(* Logix 5000 AddOnInstructionDefinition export Banner_K50Audible_Param_v4; software revision 32.00 *)

TYPE Banner_IOL_Port_v4 :   // UDT that has all of the data items necessary to communicate with a specific Port on a IO-Link Master
STRUCT
   Port_Controlled : INT;   // Each bit represents a port on an IO-Link Master. Set to 1 to tell AOI to control that port.
   Port_Activate : INT;   // Each bit represents a port on an IO-Link Master. When ON that port will process any commands in queue.
   Port_Read : INT;   // Each bit represents a port on an IO-Link Master. Used to determine when device AOI has requested a Read command.
   Port_Write : INT;   // Each bit represents a port on an IO-Link Master. Used to determine when device AOI has requested a Write command.
   Port_RW_Complete : INT;   // Each bit represents a port on an IO-Link Master. Tells device AOI that Read or Write request has been completed.
   Port_Device_Read : INT;
   Data_Transfer : SINT[190];   // Array to transfer data from IO-Master to device AOIs.
END_STRUCT
END_TYPE

TYPE Banner_K50Audible_RD_v2 :   // UDT with all of the Read only parameters for K50 Pro Audible.
STRUCT
   Master_Cycle_Time : INT;
   Min_Cycle_Time : INT;
   M_Sequence_Capability : INT;
   IO_Link_Version_ID : INT;
   Process_Data_Input_Length : INT;
   Process_Data_Output_Length : INT;
   Combined_Vendor_ID : DINT;   // IO-Link Vendor ID
   Vendor_ID1 : INT;
   Vendor_ID2 : INT;
   Combined_Device_ID : DINT;   // IO-Link Device ID
   Device_ID1 : INT;
   Device_ID2 : INT;
   Device_ID3 : INT;
   Serial_Number : STRING;
END_STRUCT
END_TYPE

TYPE Banner_K50Audible_SP_v2 :   // UDT for K50 Pro Audible Touch with the State Parameters structure.
STRUCT
   Type : SINT;   // 0 = Off, 1 = Steady, 2 = Flash, 3 = Two Color Flash, 4 = 50/50, 5 = 50/50 Rotate, 6 = Chase, 7 = Intensity Sweep, 8 = Sequence.
   Direction : SINT;   // 0 = CCW, 1 = CW.
   Pattern : SINT;   // 0 = Flash, 1 = Strobe, 2 = Three Pulse, 3 = SOS, 4 = Random.
   Speed : SINT;   // 0 = Slow, 1 = Medium, 2 = Fast, 3 = Custom.
   Audio_Feedback : SINT;   // 0 = Off, 1 = On, 2 = Animation Pattern, 3 = Advanced Audible
   Off_Delay_Type : SINT;   // 0 =Leading Edge, 1 = Trailing Edge.
   Off_Delay : DINT;   // 0 to 65535 in ms. Length of time before the device returns to 'touch inactive' state after button is released.
   Static_Sequence : INT;   // 0 to 255. Value describing the LED position of the device.
   Sequence_Start_Location : SINT;   // 0 = LED1, 1 = LED2, 2 = LED3, 3 = LED4, 4 = LED5, 5 = LED6, 6 = LED7, 7 = LED8.
   Color_1 : SINT;   // 0 = Green, 1 = Red, 2 = Orange, 3 = Amber, 4 = Yellow, 5 = Lime Green, 6 = Spring Green, 7 = Cyan, 8 = SKy Blue, 9 = Blue, 10 = Violet, 11 = Magenta, 12 = Rose, 13 = White, 14 Custom 1, 15 = Custom 2.
   Color_1_Intensity : SINT;   // 0 = High, 1 = Medium, 2 = Low, 3 = Off, 4 = Custom.
   Color_2 : SINT;   // 0 = Green, 1 = Red, 2 = Orange, 3 = Amber, 4 = Yellow, 5 = Lime Green, 6 = Spring Green, 7 = Cyan, 8 = SKy Blue, 9 = Blue, 10 = Violet, 11 = Magenta, 12 = Rose, 13 = White, 14 Custom 1, 15 = Custom 2.
   Color_2_Intensity : SINT;   // 0 = High, 1 = Medium, 2 = Low, 3 = Off, 4 = Custom.
   Audio_Volume : SINT;   // 1 = Low, 3 = High
   Audio_Type : SINT;   // 0 = Pulse, 1 = Wobble, 2 = Strobe, 3 = Whoop, 4 = Stacatto, 5 = Siren, 6 = Continuous 1, 7 = Continuous 2, 9 = Jingle, 10 = Melody 1, 11 = Melody 2, 12 = Melody 3, 13 = Custom
END_STRUCT
END_TYPE

TYPE Banner_K50Audible_v2 :   // UDT with all of the parameters for K50 Pro Audible.
STRUCT
   Initial_Global_Read : BOOL;   // Determines if all of the IO-Link data has been read into the PLC yet
   Command : INT;   // Value placed in here will activate a read or write to a specifc IO-Link Index
   Read_Data : Banner_K50Audible_RD_v2;   // All read data
   Write_Data : Banner_K50Audible_WD_v2;   // All data that can be written to.
   Archive : Banner_K50Audible_WD_v2;   // Archive of the write data.
   Reset : BOOL;
END_STRUCT
END_TYPE

TYPE Banner_K50Audible_WD_v2 :   // UDT that stores the Write Data for a K50 Pro Audible.
STRUCT
   System_Command : INT;   // See IODD file for list of commands that can be activated via the System Command interface
   Parameter_Access_Lock : SINT;   // Write access to all read/write parameters is block when this bit is ON.
   Data_Storage_Lock : SINT;   // Data storage mechanism is inhibited when bit is ON.
   Local_Parameterization_Lock : SINT;   // Parameteriation via local control elementes is inhibited.
   Local_User_Interface_Lock : SINT;   // Operation of the hmi on the device is disabled.
   Operation_Mode : SINT;   // 0 = Multicolor, 1 = Four State Full Logic, 2 = Advanced, 3 = LED Control, 4 = Demo.
   Custom_Intensity : SINT;   // 0 to 100 %
   Custom_Flash_Rate : INT;   // Range 5 to 200 (.5 to 20 converted rate).
   Restrict_to_Gamut : SINT;   // 0 = Off, 1 = On.
   Touch_Sensitivity : SINT;   // 0 = Low, 1 = High.
   Function : SINT;   // 0 = Momentary, 1 = Latched.
   Mute_Enable : SINT;   // 0 = Off, 1 = On.
   On_Delay : DINT;   // 0 to 65535 in ms. Length of time the touch button needs to be pressed to trigger touch active state.
   Output_State : SINT;   // 0 = NO, 1 = NC.
   Off_Delay_Type : SINT;   // 0 = Leading Edge, 1 = Trailing Edge.
   Off_Delay : DINT;   // 0 to 65535 in ms. Length of time before the device returns to the 'touch inactive' state after button is released.
   State_Parameters : Banner_K50Audible_SP_v2[5];   // State Parameters. 1 through 4 will have values.
   CC1_Red : INT;   // 0-255. Custom 1 Red.
   CC1_Green : INT;   // 0-255. Custom 1 Green.
   CC1_Blue : INT;   // 0-255. Custom 1 Blue.
   CC2_Red : INT;   // 0-255. Custom 2 Red.
   CC2_Green : INT;   // 0-255. Custom 2 Green.
   CC2_Blue : INT;   // 0-255. Custom 2 Blue.
   Audio_Type : SINT;   // 0 = Beep, 1 = Sweep, 2 = Tone
   Sweep_Type : SINT;   // 0 = Up, 1 = Down, 2 = Up Down, 3 = Down Up
   Freq_1 : SINT;   // 0 = Off, 1 = Low, 2 = Standard, 3 = High
   Freq_2 : SINT;   // 0 = Off, 1 = Low, 2 = Standard, 3 = High
END_STRUCT
END_TYPE

ADD_ON_INSTRUCTION Banner_K50Audible_Param_v4   (* revision 4.0, vendor Banner Engineering *)
// AOI to read and write parameter data to an IO-Link K50 Pro Audible.
VAR_IN_OUT
   K50 : Banner_K50Audible_v2; {required}
   Port_Data : Banner_IOL_Port_v4; {required}
END_VAR
VAR_INPUT
   Port : DINT; {required}
END_VAR
VAR
   Local_Control : DINT; {access None}
   Global_Read_Command_Value : INT; {access None}
   Global_Write_Command_Value : INT; {access None}
   Command_Being_Processed : BOOL; {access None}
   Update_Archive : BOOL; {access None}
   Index_Write_Control : DINT; {access None}
   Index_Write_Inprocess : INT; {access None}
   Temp_Excess_Gain : DINT[2]; {access None}
   Inprocess_Index : DINT; {access None}
   SP_Index : DINT; {access None}   // State Parameters Index
   SP_Write_Index : DINT; {access None}
   SP_R_Index : DINT; {access None}
   SP_W_Index : DINT; {access None}
END_VAR

ROUTINE Logic   (* ladder *)
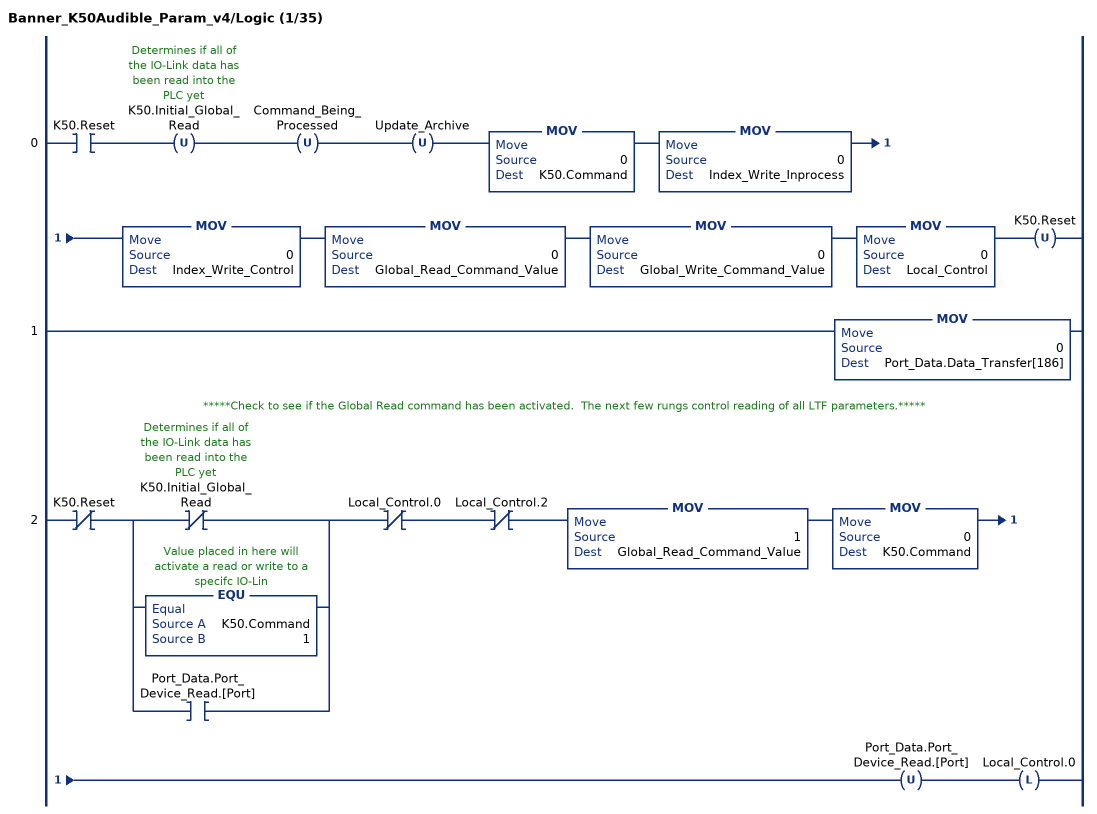
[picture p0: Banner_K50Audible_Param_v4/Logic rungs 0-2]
   0: XIC(K50.Reset)OTU(K50.Initial_Global_Read)OTU(Command_Being_Processed)OTU(Update_Archive)MOV(0,K50.Command)MOV(0,Index_Write_Inprocess)MOV(0,Index_Write_Control)MOV(0,Global_Read_Command_Value)MOV(0,Global_Write_Command_Value)MOV(0,Local_Control)OTU(K50.Reset);
   1: MOV(0,Port_Data.Data_Transfer[186]);
   // *****Check to see if the Global Read command has been activated.  The next few rungs control reading of all LTF parameters.*****
   2: XIO(K50.Reset)[XIO(K50.Initial_Global_Read) ,EQU(K50.Command,1) ,XIC(Port_Data.Port_Device_Read.[Port]) ]XIO(Local_Control.0)XIO(Local_Control.2)MOV(1,Global_Read_Command_Value)MOV(0,K50.Command)OTU(Port_Data.Port_Device_Read.[Port])OTL(Local_Control.0);
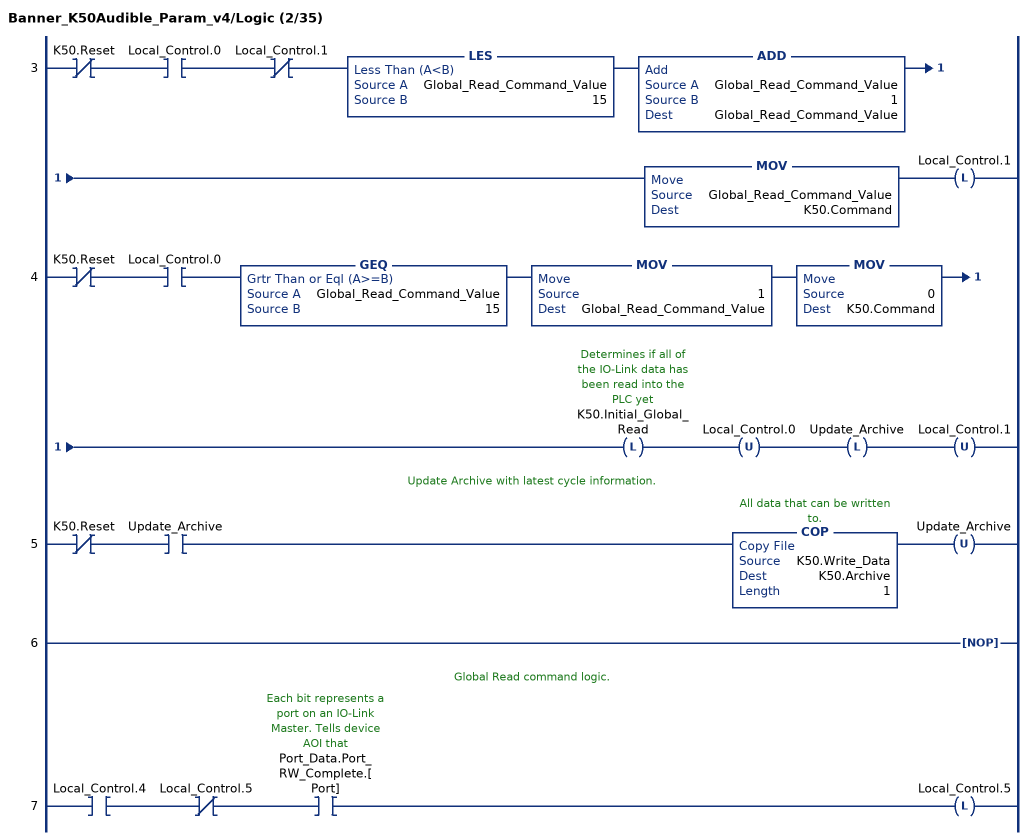
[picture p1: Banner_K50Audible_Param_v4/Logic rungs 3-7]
   3: XIO(K50.Reset)XIC(Local_Control.0)XIO(Local_Control.1)LES(Global_Read_Command_Value,15)ADD(Global_Read_Command_Value,1,Global_Read_Command_Value)MOV(Global_Read_Command_Value,K50.Command)OTL(Local_Control.1);
   4: XIO(K50.Reset)XIC(Local_Control.0)GEQ(Global_Read_Command_Value,15)MOV(1,Global_Read_Command_Value)MOV(0,K50.Command)OTL(K50.Initial_Global_Read)OTU(Local_Control.0)OTL(Update_Archive)OTU(Local_Control.1);
   // Update Archive with latest cycle information.
   5: XIO(K50.Reset)XIC(Update_Archive)COP(K50.Write_Data,K50.Archive,1)OTU(Update_Archive);
   6: NOP();
   // Global Read command logic.
   7: XIC(Local_Control.4)XIO(Local_Control.5)XIC(Port_Data.Port_RW_Complete.[Port])OTL(Local_Control.5);
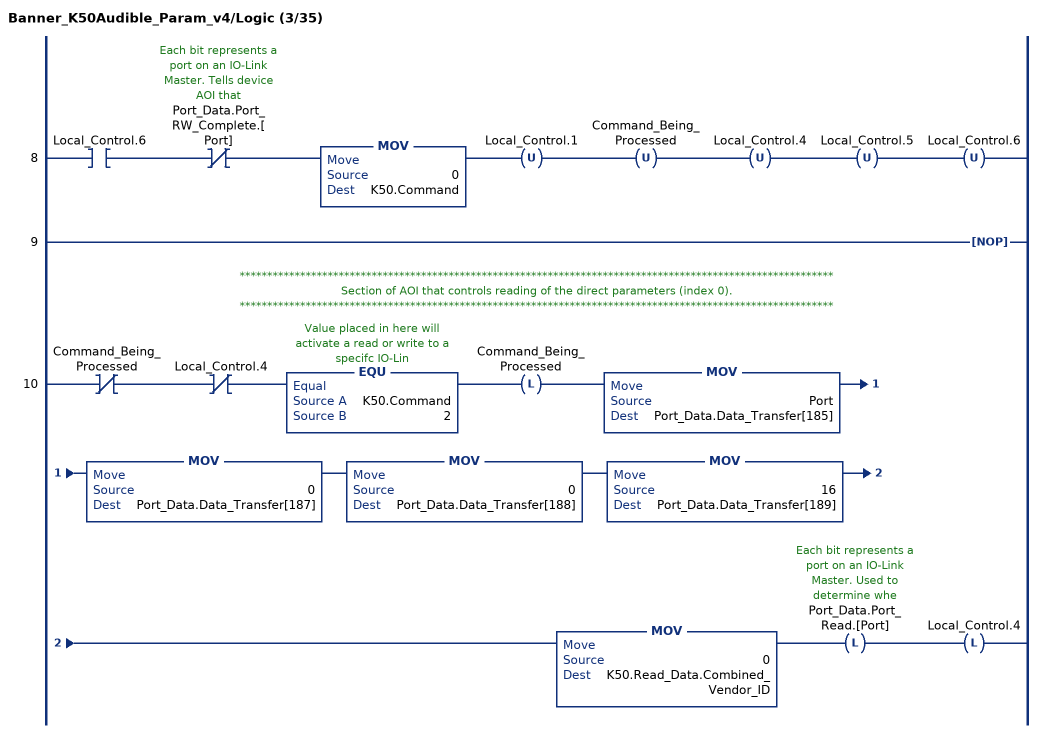
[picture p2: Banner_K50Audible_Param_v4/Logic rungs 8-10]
   8: XIC(Local_Control.6)XIO(Port_Data.Port_RW_Complete.[Port])MOV(0,K50.Command)OTU(Local_Control.1)OTU(Command_Being_Processed)OTU(Local_Control.4)OTU(Local_Control.5)OTU(Local_Control.6);
   9: NOP();
   // ************************************************************************************************************
   // Section of AOI that controls reading of the direct parameters (index 0).
   // ************************************************************************************************************
   10: XIO(Command_Being_Processed)XIO(Local_Control.4)EQU(K50.Command,2)OTL(Command_Being_Processed)MOV(Port,Port_Data.Data_Transfer[185])MOV(0,Port_Data.Data_Transfer[187])MOV(0,Port_Data.Data_Transfer[188])MOV(16,Port_Data.Data_Transfer[189])MOV(0,K50.Read_Data.Combined_Vendor_ID)OTL(Port_Data.Port_Read.[Port])OTL(Local_Control.4);
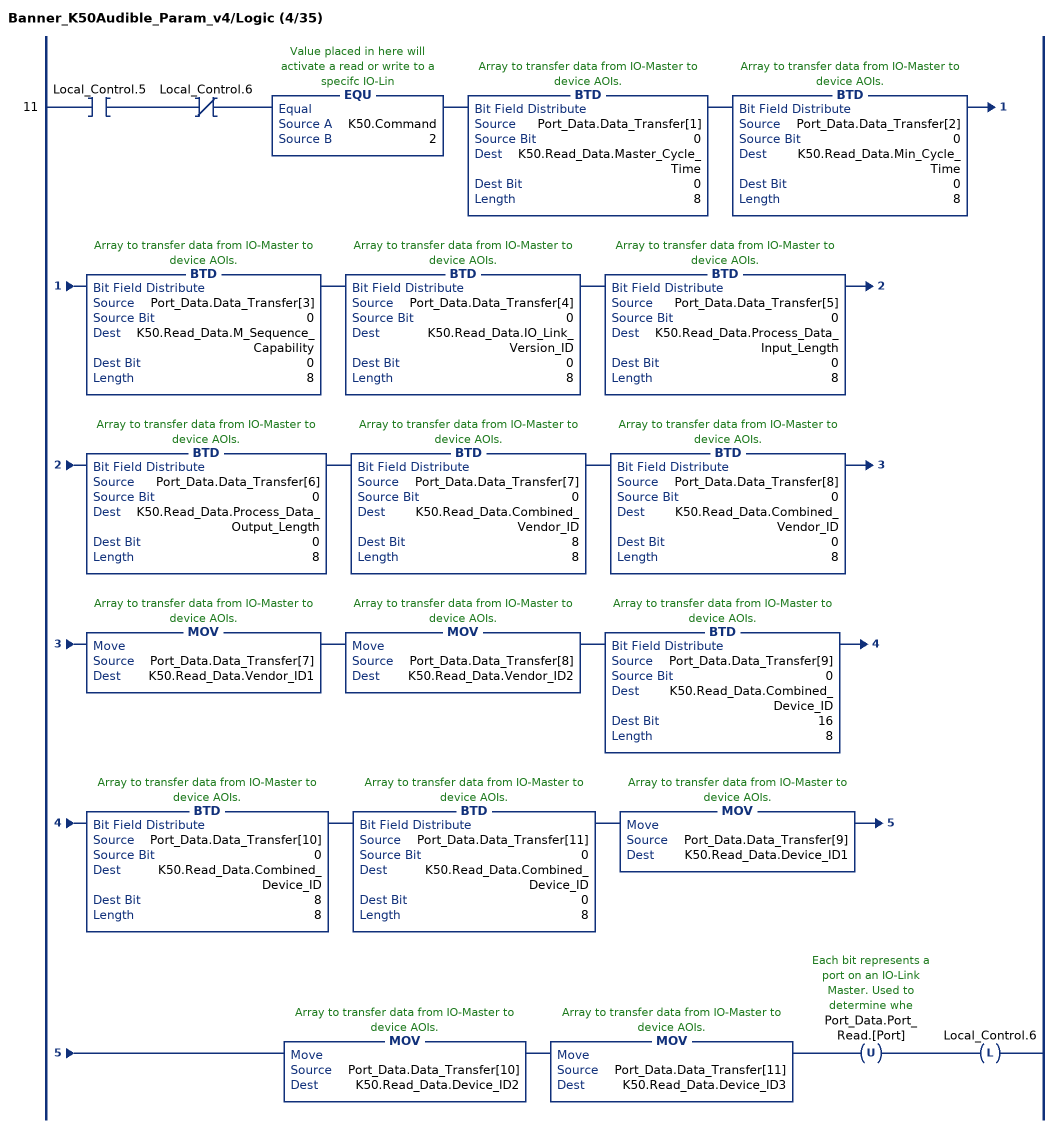
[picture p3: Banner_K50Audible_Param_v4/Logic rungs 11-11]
   11: XIC(Local_Control.5)XIO(Local_Control.6)EQU(K50.Command,2)BTD(Port_Data.Data_Transfer[1],0,K50.Read_Data.Master_Cycle_Time,0,8)BTD(Port_Data.Data_Transfer[2],0,K50.Read_Data.Min_Cycle_Time,0,8)BTD(Port_Data.Data_Transfer[3],0,K50.Read_Data.M_Sequence_Capability,0,8)BTD(Port_Data.Data_Transfer[4],0,K50.Read_Data.IO_Link_Version_ID,0,8)BTD(Port_Data.Data_Transfer[5],0,K50.Read_Data.Process_Data_Input_Length,0,8)BTD(Port_Data.Data_Transfer[6],0,K50.Read_Data.Process_Data_Output_Length,0,8)BTD(Port_Data.Data_Transfer[7],0,K50.Read_Data.Combined_Vendor_ID,8,8)BTD(Port_Data.Data_Transfer[8],0,K50.Read_Data.Combined_Vendor_ID,0,8)MOV(Port_Data.Data_Transfer[7],K50.Read_Data.Vendor_ID1)MOV(Port_Data.Data_Transfer[8],K50.Read_Data.Vendor_ID2)BTD(Port_Data.Data_Transfer[9],0,K50.Read_Data.Combined_Device_ID,16,8)BTD(Port_Data.Data_Transfer[10],0,K50.Read_Data.Combined_Device_ID,8,8)BTD(Port_Data.Data_Transfer[11],0,K50.Read_Data.Combined_Device_ID,0,8)MOV(Port_Data.Data_Transfer[9],K50.Read_Data.Device_ID1)MOV(Port_Data.Data_Transfer[10],K50.Read_Data.Device_ID2)MOV(Port_Data.Data_Transfer[11],K50.Read_Data.Device_ID3)OTU(Port_Data.Port_Read.[Port])OTL(Local_Control.6);
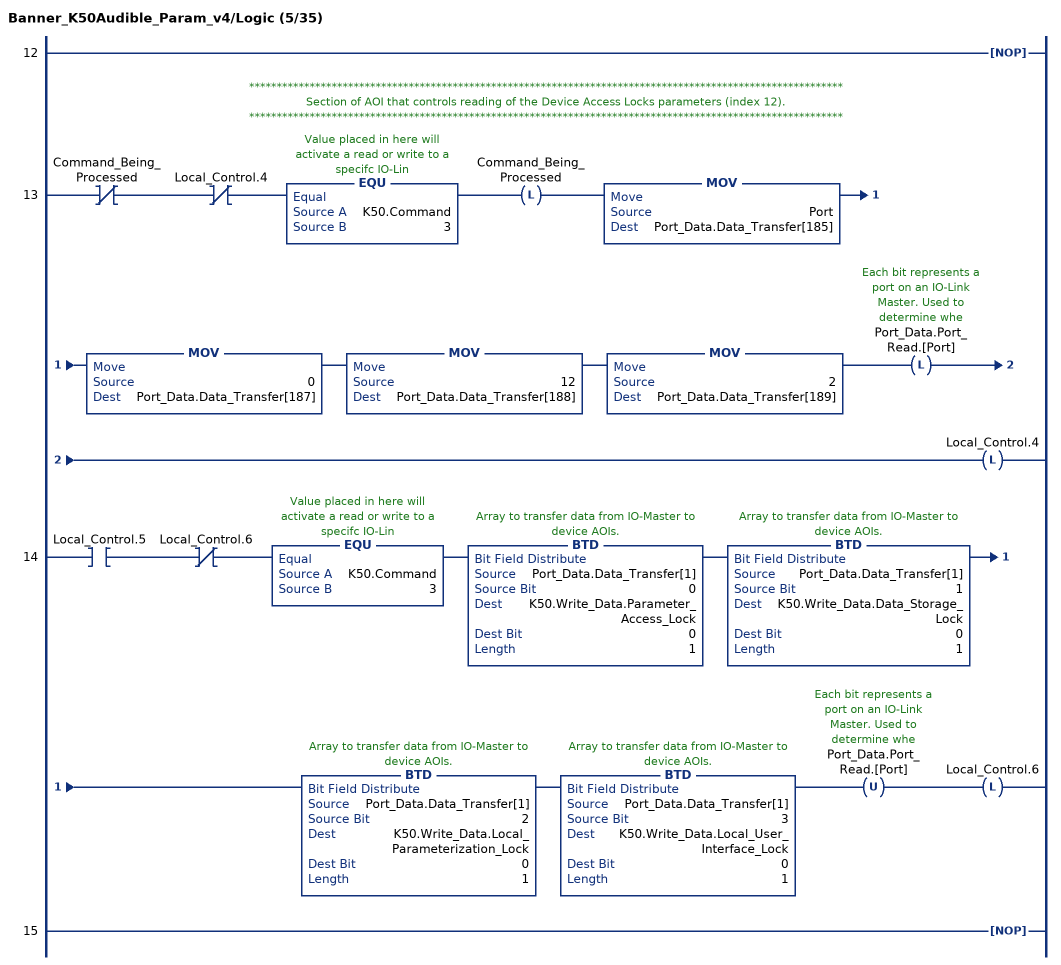
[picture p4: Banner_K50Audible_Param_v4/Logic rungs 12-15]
   12: NOP();
   // ************************************************************************************************************
   // Section of AOI that controls reading of the Device Access Locks parameters (index 12).
   // ************************************************************************************************************
   13: XIO(Command_Being_Processed)XIO(Local_Control.4)EQU(K50.Command,3)OTL(Command_Being_Processed)MOV(Port,Port_Data.Data_Transfer[185])MOV(0,Port_Data.Data_Transfer[187])MOV(12,Port_Data.Data_Transfer[188])MOV(2,Port_Data.Data_Transfer[189])OTL(Port_Data.Port_Read.[Port])OTL(Local_Control.4);
   14: XIC(Local_Control.5)XIO(Local_Control.6)EQU(K50.Command,3)BTD(Port_Data.Data_Transfer[1],0,K50.Write_Data.Parameter_Access_Lock,0,1)BTD(Port_Data.Data_Transfer[1],1,K50.Write_Data.Data_Storage_Lock,0,1)BTD(Port_Data.Data_Transfer[1],2,K50.Write_Data.Local_Parameterization_Lock,0,1)BTD(Port_Data.Data_Transfer[1],3,K50.Write_Data.Local_User_Interface_Lock,0,1)OTU(Port_Data.Port_Read.[Port])OTL(Local_Control.6);
   15: NOP();
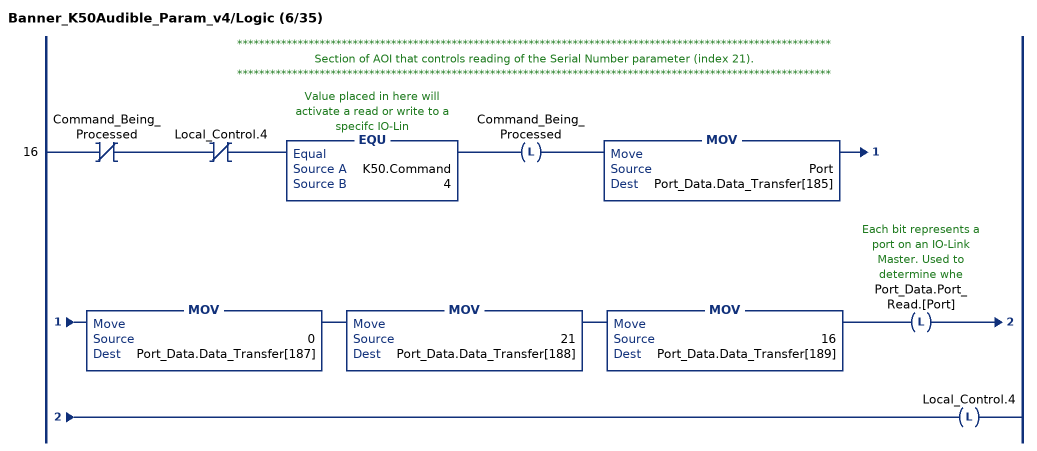
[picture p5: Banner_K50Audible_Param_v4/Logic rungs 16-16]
   // ************************************************************************************************************
   // Section of AOI that controls reading of the Serial Number parameter (index 21).
   // ************************************************************************************************************
   16: XIO(Command_Being_Processed)XIO(Local_Control.4)EQU(K50.Command,4)OTL(Command_Being_Processed)MOV(Port,Port_Data.Data_Transfer[185])MOV(0,Port_Data.Data_Transfer[187])MOV(21,Port_Data.Data_Transfer[188])MOV(16,Port_Data.Data_Transfer[189])OTL(Port_Data.Port_Read.[Port])OTL(Local_Control.4);
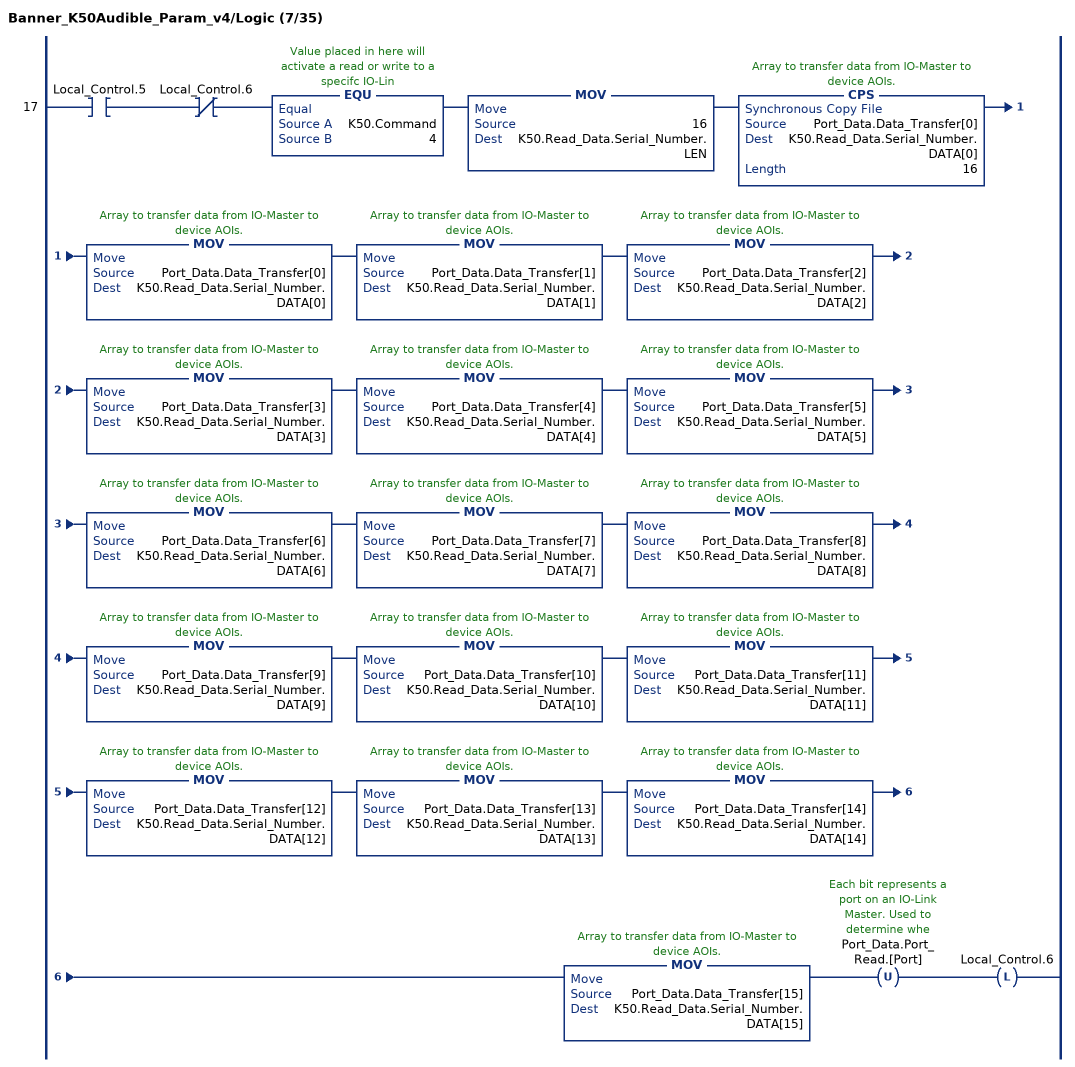
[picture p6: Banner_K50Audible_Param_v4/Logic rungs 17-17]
   17: XIC(Local_Control.5)XIO(Local_Control.6)EQU(K50.Command,4)MOV(16,K50.Read_Data.Serial_Number.LEN)CPS(Port_Data.Data_Transfer[0],K50.Read_Data.Serial_Number.DATA[0],16)MOV(Port_Data.Data_Transfer[0],K50.Read_Data.Serial_Number.DATA[0])MOV(Port_Data.Data_Transfer[1],K50.Read_Data.Serial_Number.DATA[1])MOV(Port_Data.Data_Transfer[2],K50.Read_Data.Serial_Number.DATA[2])MOV(Port_Data.Data_Transfer[3],K50.Read_Data.Serial_Number.DATA[3])MOV(Port_Data.Data_Transfer[4],K50.Read_Data.Serial_Number.DATA[4])MOV(Port_Data.Data_Transfer[5],K50.Read_Data.Serial_Number.DATA[5])MOV(Port_Data.Data_Transfer[6],K50.Read_Data.Serial_Number.DATA[6])MOV(Port_Data.Data_Transfer[7],K50.Read_Data.Serial_Number.DATA[7])MOV(Port_Data.Data_Transfer[8],K50.Read_Data.Serial_Number.DATA[8])MOV(Port_Data.Data_Transfer[9],K50.Read_Data.Serial_Number.DATA[9])MOV(Port_Data.Data_Transfer[10],K50.Read_Data.Serial_Number.DATA[10])MOV(Port_Data.Data_Transfer[11],K50.Read_Data.Serial_Number.DATA[11])MOV(Port_Data.Data_Transfer[12],K50.Read_Data.Serial_Number.DATA[12])MOV(Port_Data.Data_Transfer[13],K50.Read_Data.Serial_Number.DATA[13])MOV(Port_Data.Data_Transfer[14],K50.Read_Data.Serial_Number.DATA[14])MOV(Port_Data.Data_Transfer[15],K50.Read_Data.Serial_Number.DATA[15])OTU(Port_Data.Port_Read.[Port])OTL(Local_Control.6);
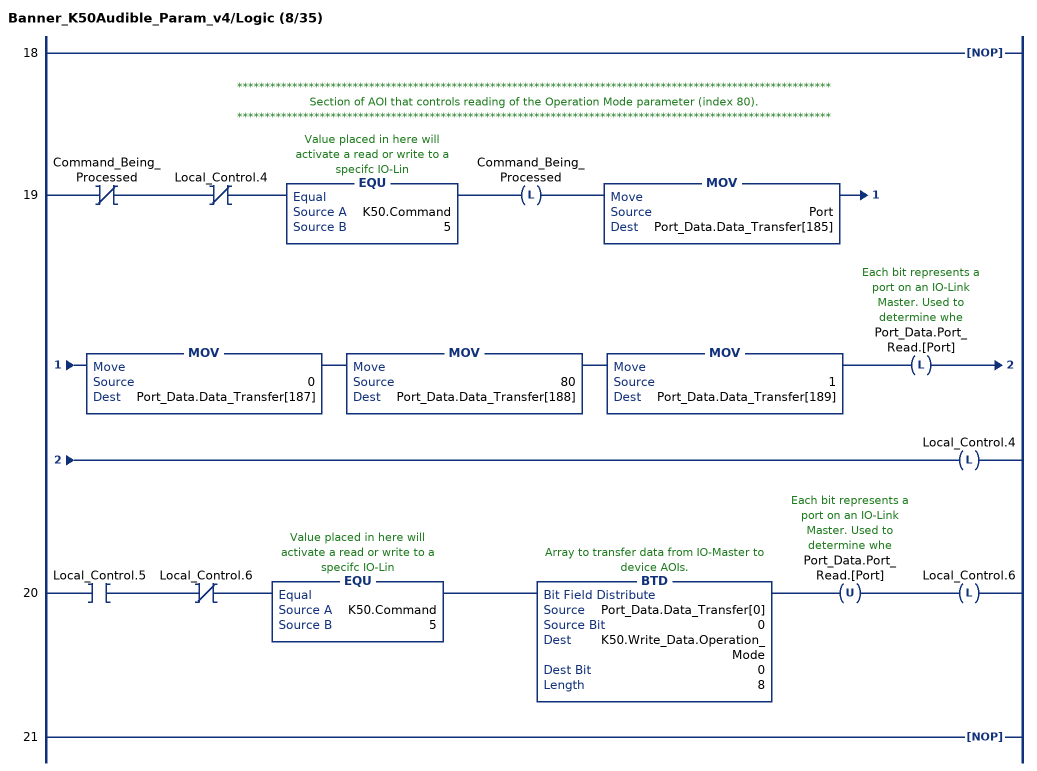
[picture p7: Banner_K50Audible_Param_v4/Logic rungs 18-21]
   18: NOP();
   // ************************************************************************************************************
   // Section of AOI that controls reading of the Operation Mode parameter (index 80).
   // ************************************************************************************************************
   19: XIO(Command_Being_Processed)XIO(Local_Control.4)EQU(K50.Command,5)OTL(Command_Being_Processed)MOV(Port,Port_Data.Data_Transfer[185])MOV(0,Port_Data.Data_Transfer[187])MOV(80,Port_Data.Data_Transfer[188])MOV(1,Port_Data.Data_Transfer[189])OTL(Port_Data.Port_Read.[Port])OTL(Local_Control.4);
   20: XIC(Local_Control.5)XIO(Local_Control.6)EQU(K50.Command,5)BTD(Port_Data.Data_Transfer[0],0,K50.Write_Data.Operation_Mode,0,8)OTU(Port_Data.Port_Read.[Port])OTL(Local_Control.6);
   21: NOP();
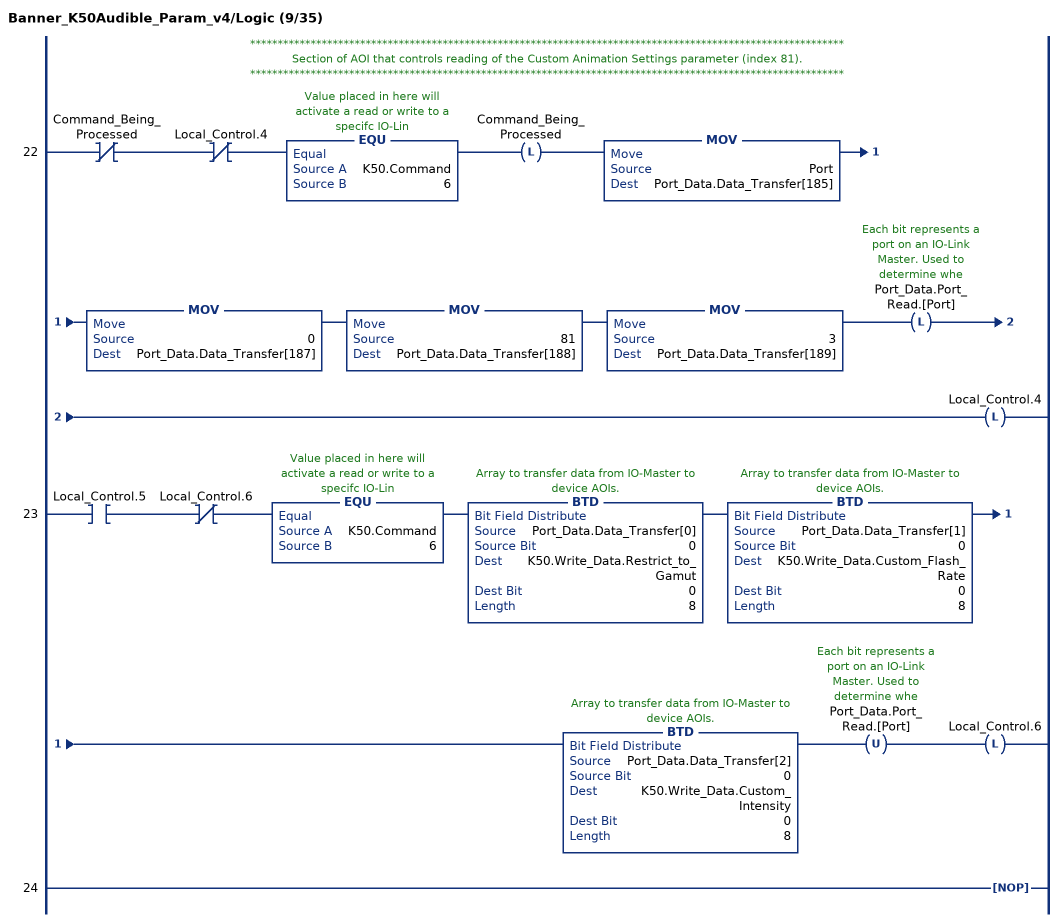
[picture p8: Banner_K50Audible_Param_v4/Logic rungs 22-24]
   // ************************************************************************************************************
   // Section of AOI that controls reading of the Custom Animation Settings parameter (index 81).
   // ************************************************************************************************************
   22: XIO(Command_Being_Processed)XIO(Local_Control.4)EQU(K50.Command,6)OTL(Command_Being_Processed)MOV(Port,Port_Data.Data_Transfer[185])MOV(0,Port_Data.Data_Transfer[187])MOV(81,Port_Data.Data_Transfer[188])MOV(3,Port_Data.Data_Transfer[189])OTL(Port_Data.Port_Read.[Port])OTL(Local_Control.4);
   23: XIC(Local_Control.5)XIO(Local_Control.6)EQU(K50.Command,6)BTD(Port_Data.Data_Transfer[0],0,K50.Write_Data.Restrict_to_Gamut,0,8)BTD(Port_Data.Data_Transfer[1],0,K50.Write_Data.Custom_Flash_Rate,0,8)BTD(Port_Data.Data_Transfer[2],0,K50.Write_Data.Custom_Intensity,0,8)OTU(Port_Data.Port_Read.[Port])OTL(Local_Control.6);
   24: NOP();
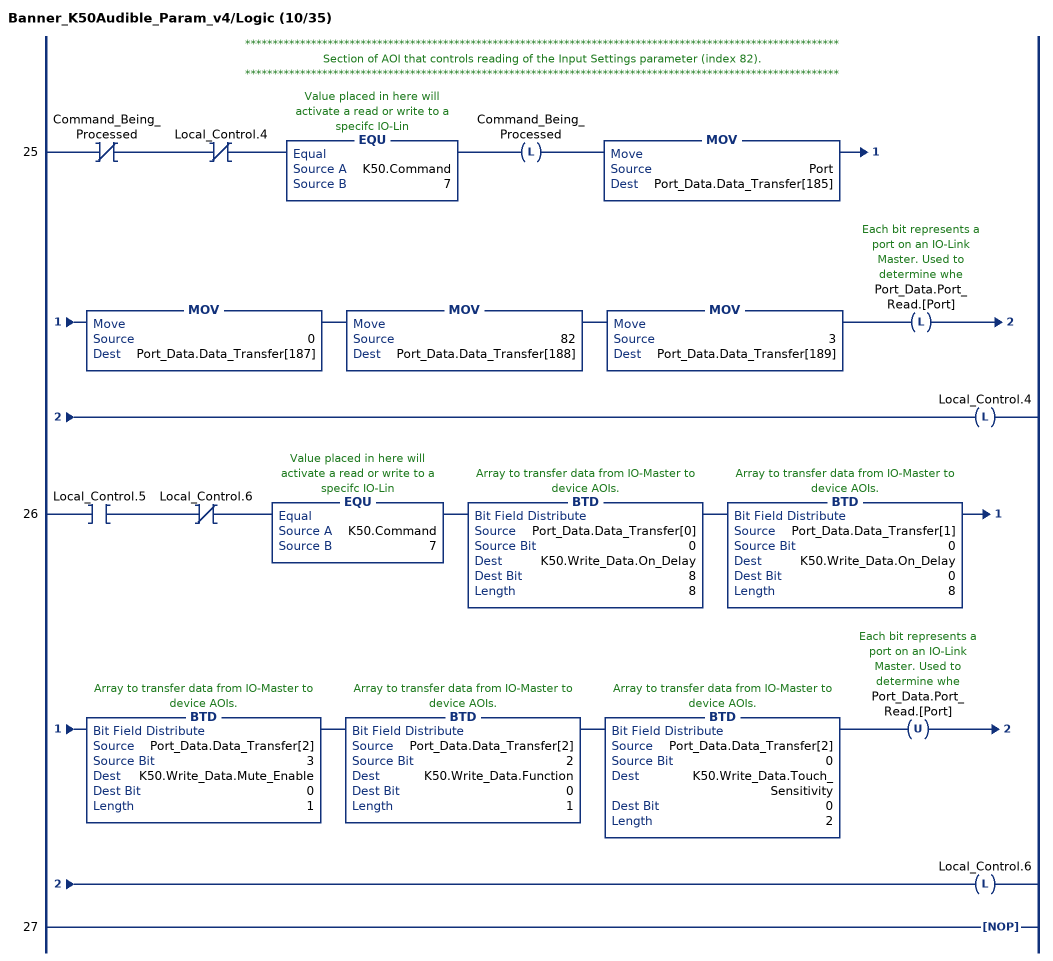
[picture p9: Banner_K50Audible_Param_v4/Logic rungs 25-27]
   // ************************************************************************************************************
   // Section of AOI that controls reading of the Input Settings parameter (index 82).
   // ************************************************************************************************************
   25: XIO(Command_Being_Processed)XIO(Local_Control.4)EQU(K50.Command,7)OTL(Command_Being_Processed)MOV(Port,Port_Data.Data_Transfer[185])MOV(0,Port_Data.Data_Transfer[187])MOV(82,Port_Data.Data_Transfer[188])MOV(3,Port_Data.Data_Transfer[189])OTL(Port_Data.Port_Read.[Port])OTL(Local_Control.4);
   26: XIC(Local_Control.5)XIO(Local_Control.6)EQU(K50.Command,7)BTD(Port_Data.Data_Transfer[0],0,K50.Write_Data.On_Delay,8,8)BTD(Port_Data.Data_Transfer[1],0,K50.Write_Data.On_Delay,0,8)BTD(Port_Data.Data_Transfer[2],3,K50.Write_Data.Mute_Enable,0,1)BTD(Port_Data.Data_Transfer[2],2,K50.Write_Data.Function,0,1)BTD(Port_Data.Data_Transfer[2],0,K50.Write_Data.Touch_Sensitivity,0,2)OTU(Port_Data.Port_Read.[Port])OTL(Local_Control.6);
   27: NOP();
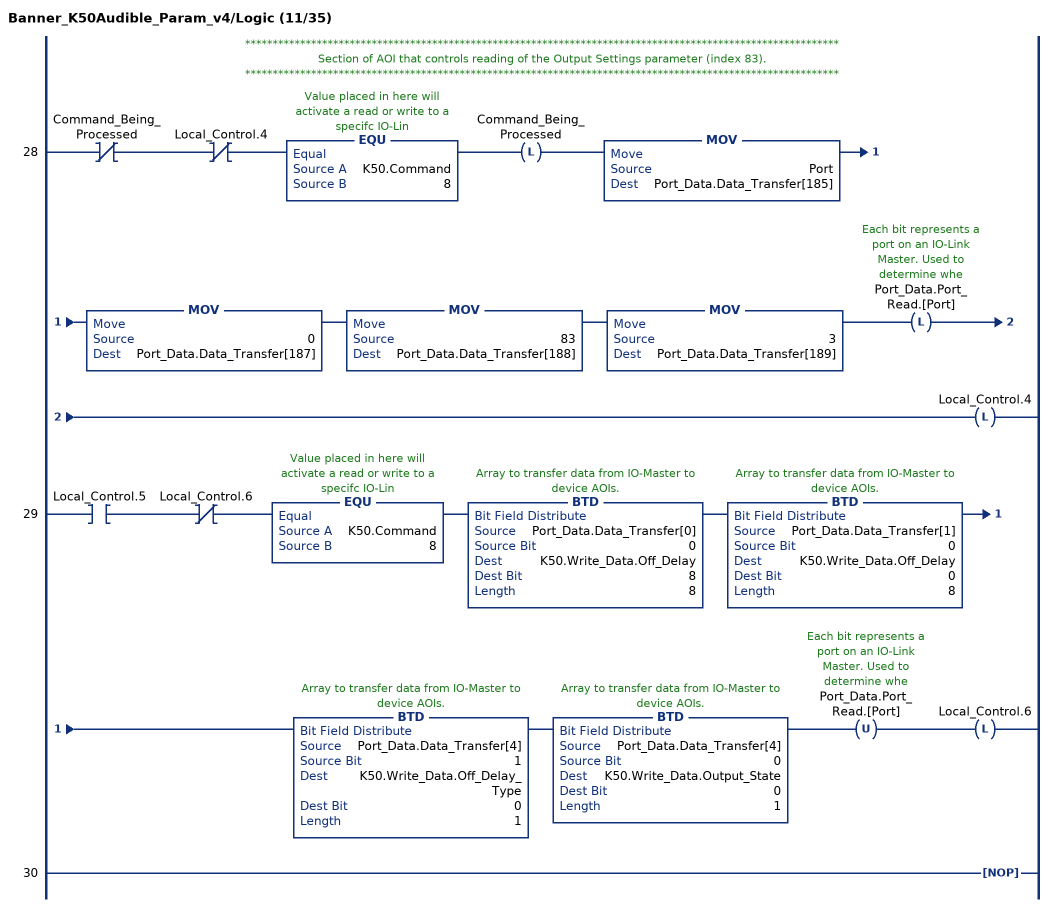
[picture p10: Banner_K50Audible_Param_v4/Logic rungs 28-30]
   // ************************************************************************************************************
   // Section of AOI that controls reading of the Output Settings parameter (index 83).
   // ************************************************************************************************************
   28: XIO(Command_Being_Processed)XIO(Local_Control.4)EQU(K50.Command,8)OTL(Command_Being_Processed)MOV(Port,Port_Data.Data_Transfer[185])MOV(0,Port_Data.Data_Transfer[187])MOV(83,Port_Data.Data_Transfer[188])MOV(3,Port_Data.Data_Transfer[189])OTL(Port_Data.Port_Read.[Port])OTL(Local_Control.4);
   29: XIC(Local_Control.5)XIO(Local_Control.6)EQU(K50.Command,8)BTD(Port_Data.Data_Transfer[0],0,K50.Write_Data.Off_Delay,8,8)BTD(Port_Data.Data_Transfer[1],0,K50.Write_Data.Off_Delay,0,8)BTD(Port_Data.Data_Transfer[4],1,K50.Write_Data.Off_Delay_Type,0,1)BTD(Port_Data.Data_Transfer[4],0,K50.Write_Data.Output_State,0,1)OTU(Port_Data.Port_Read.[Port])OTL(Local_Control.6);
   30: NOP();
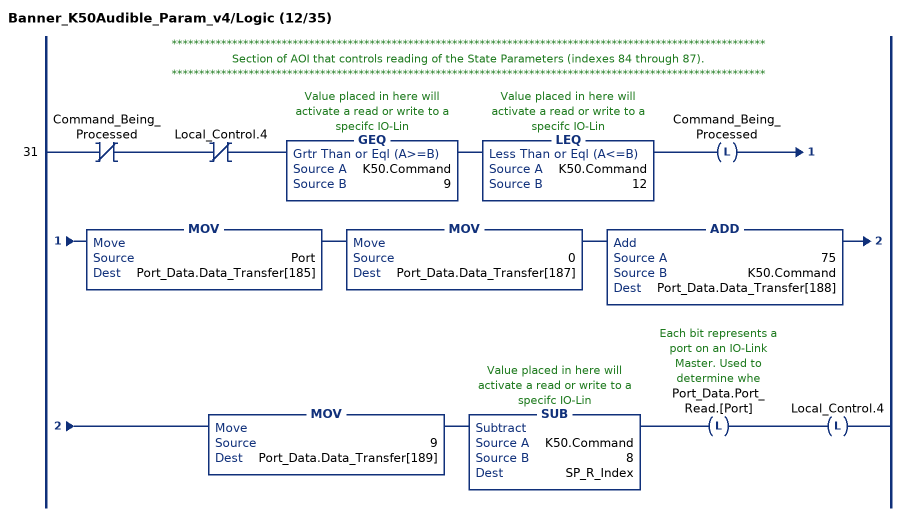
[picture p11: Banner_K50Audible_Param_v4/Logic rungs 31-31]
   // ************************************************************************************************************
   // Section of AOI that controls reading of the State Parameters (indexes 84 through 87).
   // ************************************************************************************************************
   31: XIO(Command_Being_Processed)XIO(Local_Control.4)GEQ(K50.Command,9)LEQ(K50.Command,12)OTL(Command_Being_Processed)MOV(Port,Port_Data.Data_Transfer[185])MOV(0,Port_Data.Data_Transfer[187])ADD(75,K50.Command,Port_Data.Data_Transfer[188])MOV(9,Port_Data.Data_Transfer[189])SUB(K50.Command,8,SP_R_Index)OTL(Port_Data.Port_Read.[Port])OTL(Local_Control.4);
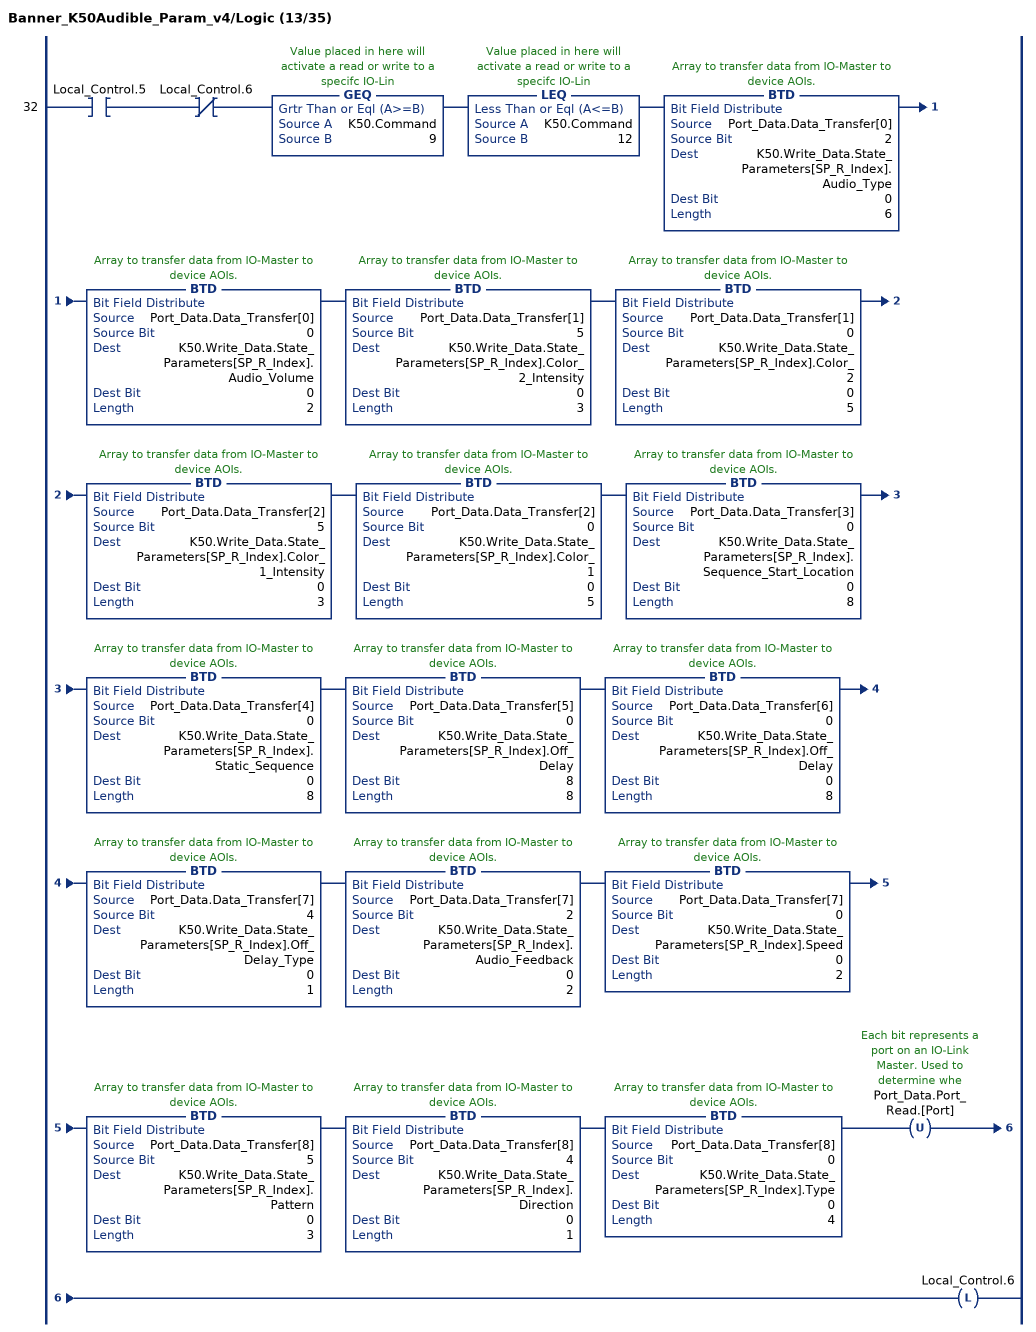
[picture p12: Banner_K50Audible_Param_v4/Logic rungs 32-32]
   32: XIC(Local_Control.5)XIO(Local_Control.6)GEQ(K50.Command,9)LEQ(K50.Command,12)BTD(Port_Data.Data_Transfer[0],2,K50.Write_Data.State_Parameters[SP_R_Index].Audio_Type,0,6)BTD(Port_Data.Data_Transfer[0],0,K50.Write_Data.State_Parameters[SP_R_Index].Audio_Volume,0,2)BTD(Port_Data.Data_Transfer[1],5,K50.Write_Data.State_Parameters[SP_R_Index].Color_2_Intensity,0,3)BTD(Port_Data.Data_Transfer[1],0,K50.Write_Data.State_Parameters[SP_R_Index].Color_2,0,5)BTD(Port_Data.Data_Transfer[2],5,K50.Write_Data.State_Parameters[SP_R_Index].Color_1_Intensity,0,3)BTD(Port_Data.Data_Transfer[2],0,K50.Write_Data.State_Parameters[SP_R_Index].Color_1,0,5)BTD(Port_Data.Data_Transfer[3],0,K50.Write_Data.State_Parameters[SP_R_Index].Sequence_Start_Location,0,8)BTD(Port_Data.Data_Transfer[4],0,K50.Write_Data.State_Parameters[SP_R_Index].Static_Sequence,0,8)BTD(Port_Data.Data_Transfer[5],0,K50.Write_Data.State_Parameters[SP_R_Index].Off_Delay,8,8)BTD(Port_Data.Data_Transfer[6],0,K50.Write_Data.State_Parameters[SP_R_Index].Off_Delay,0,8)BTD(Port_Data.Data_Transfer[7],4,K50.Write_Data.State_Parameters[SP_R_Index].Off_Delay_Type,0,1)BTD(Port_Data.Data_Transfer[7],2,K50.Write_Data.State_Parameters[SP_R_Index].Audio_Feedback,0,2)BTD(Port_Data.Data_Transfer[7],0,K50.Write_Data.State_Parameters[SP_R_Index].Speed,0,2)BTD(Port_Data.Data_Transfer[8],5,K50.Write_Data.State_Parameters[SP_R_Index].Pattern,0,3)BTD(Port_Data.Data_Transfer[8],4,K50.Write_Data.State_Parameters[SP_R_Index].Direction,0,1)BTD(Port_Data.Data_Transfer[8],0,K50.Write_Data.State_Parameters[SP_R_Index].Type,0,4)OTU(Port_Data.Port_Read.[Port])OTL(Local_Control.6);
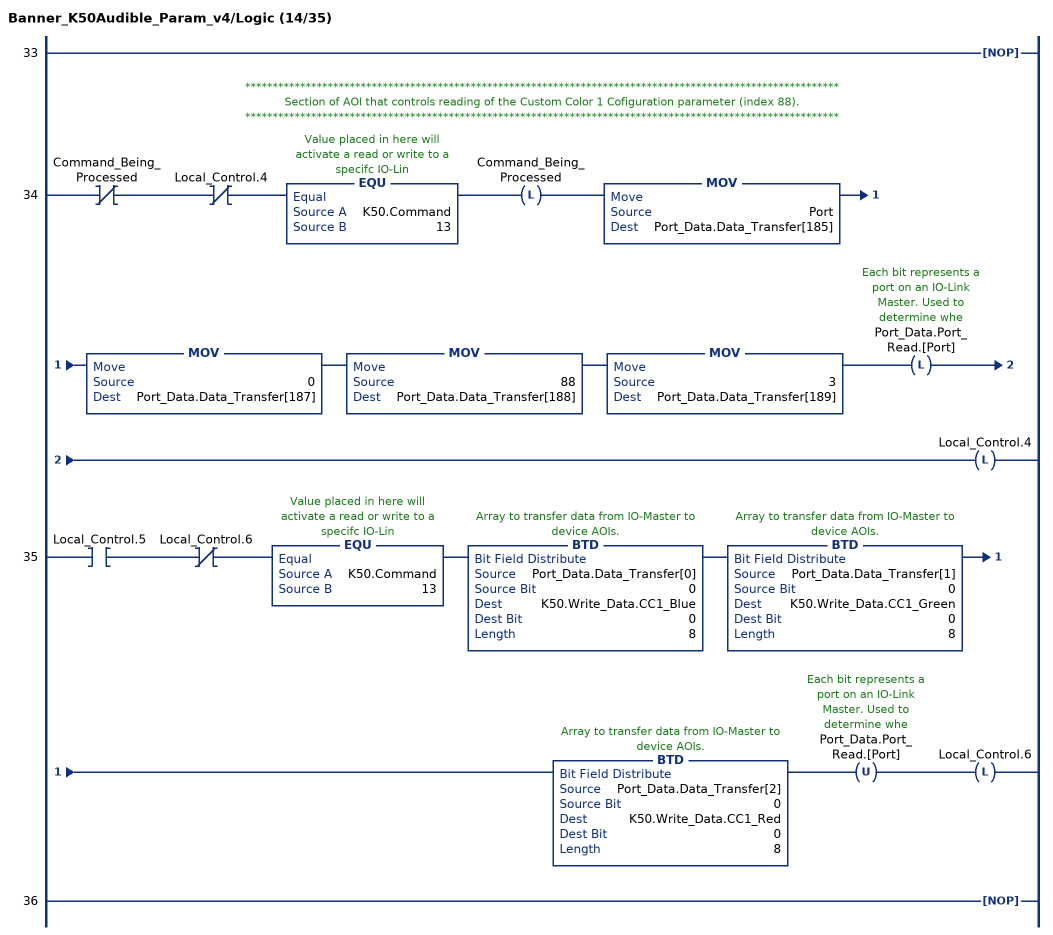
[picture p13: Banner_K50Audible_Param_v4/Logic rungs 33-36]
   33: NOP();
   // ************************************************************************************************************
   // Section of AOI that controls reading of the Custom Color 1 Cofiguration parameter (index 88).
   // ************************************************************************************************************
   34: XIO(Command_Being_Processed)XIO(Local_Control.4)EQU(K50.Command,13)OTL(Command_Being_Processed)MOV(Port,Port_Data.Data_Transfer[185])MOV(0,Port_Data.Data_Transfer[187])MOV(88,Port_Data.Data_Transfer[188])MOV(3,Port_Data.Data_Transfer[189])OTL(Port_Data.Port_Read.[Port])OTL(Local_Control.4);
   35: XIC(Local_Control.5)XIO(Local_Control.6)EQU(K50.Command,13)BTD(Port_Data.Data_Transfer[0],0,K50.Write_Data.CC1_Blue,0,8)BTD(Port_Data.Data_Transfer[1],0,K50.Write_Data.CC1_Green,0,8)BTD(Port_Data.Data_Transfer[2],0,K50.Write_Data.CC1_Red,0,8)OTU(Port_Data.Port_Read.[Port])OTL(Local_Control.6);
   36: NOP();
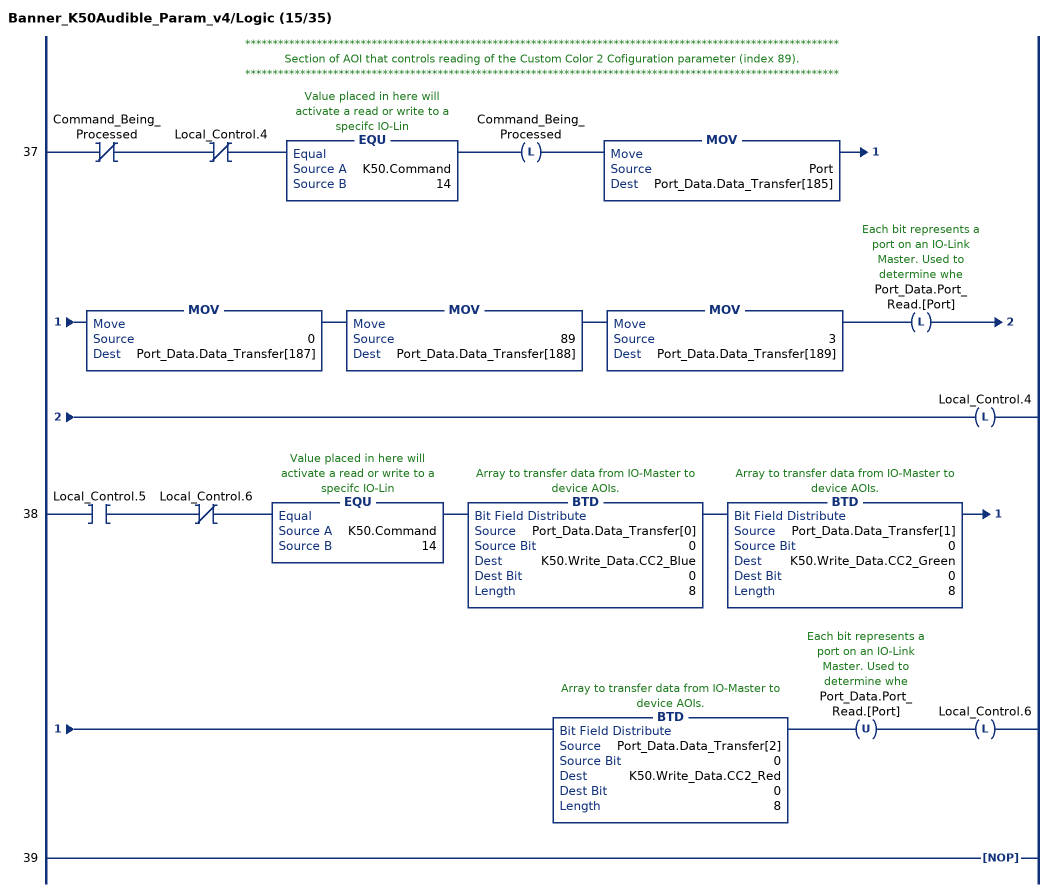
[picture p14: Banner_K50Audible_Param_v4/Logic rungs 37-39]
   // ************************************************************************************************************
   // Section of AOI that controls reading of the Custom Color 2 Cofiguration parameter (index 89).
   // ************************************************************************************************************
   37: XIO(Command_Being_Processed)XIO(Local_Control.4)EQU(K50.Command,14)OTL(Command_Being_Processed)MOV(Port,Port_Data.Data_Transfer[185])MOV(0,Port_Data.Data_Transfer[187])MOV(89,Port_Data.Data_Transfer[188])MOV(3,Port_Data.Data_Transfer[189])OTL(Port_Data.Port_Read.[Port])OTL(Local_Control.4);
   38: XIC(Local_Control.5)XIO(Local_Control.6)EQU(K50.Command,14)BTD(Port_Data.Data_Transfer[0],0,K50.Write_Data.CC2_Blue,0,8)BTD(Port_Data.Data_Transfer[1],0,K50.Write_Data.CC2_Green,0,8)BTD(Port_Data.Data_Transfer[2],0,K50.Write_Data.CC2_Red,0,8)OTU(Port_Data.Port_Read.[Port])OTL(Local_Control.6);
   39: NOP();
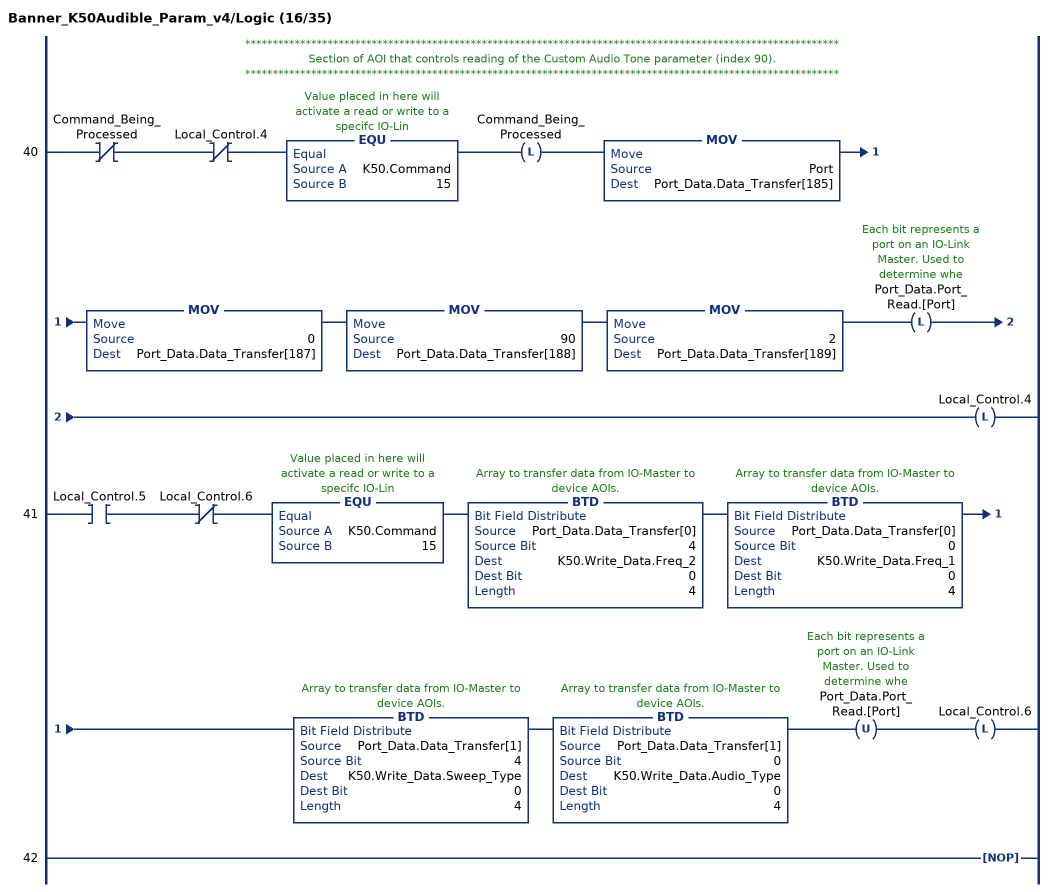
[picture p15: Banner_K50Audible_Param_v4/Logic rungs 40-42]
   // ************************************************************************************************************
   // Section of AOI that controls reading of the Custom Audio Tone parameter (index 90).
   // ************************************************************************************************************
   40: XIO(Command_Being_Processed)XIO(Local_Control.4)EQU(K50.Command,15)OTL(Command_Being_Processed)MOV(Port,Port_Data.Data_Transfer[185])MOV(0,Port_Data.Data_Transfer[187])MOV(90,Port_Data.Data_Transfer[188])MOV(2,Port_Data.Data_Transfer[189])OTL(Port_Data.Port_Read.[Port])OTL(Local_Control.4);
   41: XIC(Local_Control.5)XIO(Local_Control.6)EQU(K50.Command,15)BTD(Port_Data.Data_Transfer[0],4,K50.Write_Data.Freq_2,0,4)BTD(Port_Data.Data_Transfer[0],0,K50.Write_Data.Freq_1,0,4)BTD(Port_Data.Data_Transfer[1],4,K50.Write_Data.Sweep_Type,0,4)BTD(Port_Data.Data_Transfer[1],0,K50.Write_Data.Audio_Type,0,4)OTU(Port_Data.Port_Read.[Port])OTL(Local_Control.6);
   42: NOP();
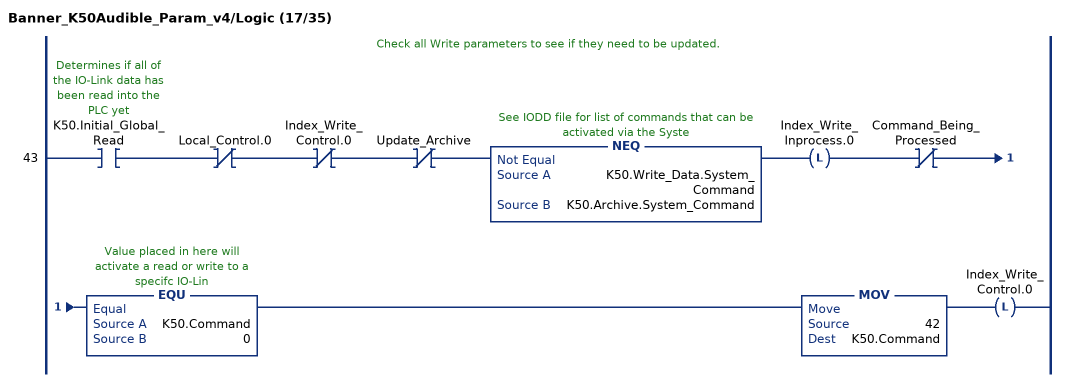
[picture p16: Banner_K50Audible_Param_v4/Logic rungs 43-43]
   // Check all Write parameters to see if they need to be updated.
   43: XIC(K50.Initial_Global_Read)XIO(Local_Control.0)XIO(Index_Write_Control.0)XIO(Update_Archive)NEQ(K50.Write_Data.System_Command,K50.Archive.System_Command)OTL(Index_Write_Inprocess.0)XIO(Command_Being_Processed)EQU(K50.Command,0)MOV(42,K50.Command)OTL(Index_Write_Control.0);
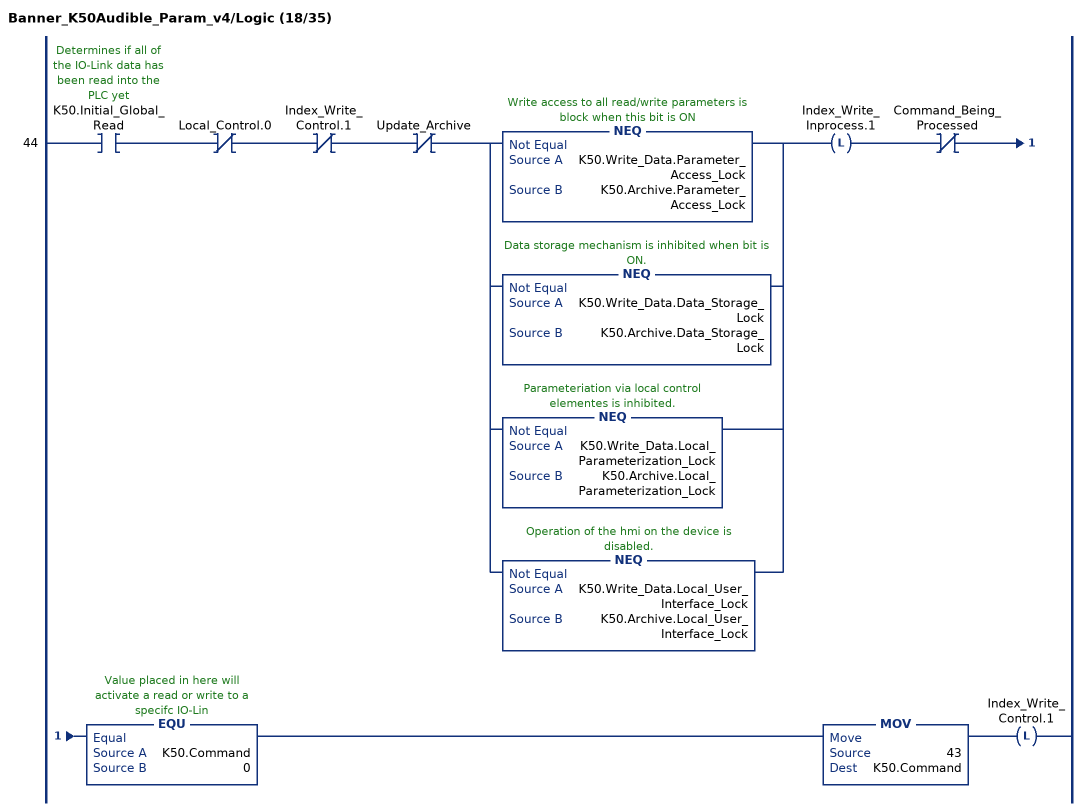
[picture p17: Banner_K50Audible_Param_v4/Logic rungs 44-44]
   44: XIC(K50.Initial_Global_Read)XIO(Local_Control.0)XIO(Index_Write_Control.1)XIO(Update_Archive)[NEQ(K50.Write_Data.Parameter_Access_Lock,K50.Archive.Parameter_Access_Lock) ,NEQ(K50.Write_Data.Data_Storage_Lock,K50.Archive.Data_Storage_Lock) ,NEQ(K50.Write_Data.Local_Parameterization_Lock,K50.Archive.Local_Parameterization_Lock) ,NEQ(K50.Write_Data.Local_User_Interface_Lock,K50.Archive.Local_User_Interface_Lock) ]OTL(Index_Write_Inprocess.1)XIO(Command_Being_Processed)EQU(K50.Command,0)MOV(43,K50.Command)OTL(Index_Write_Control.1);
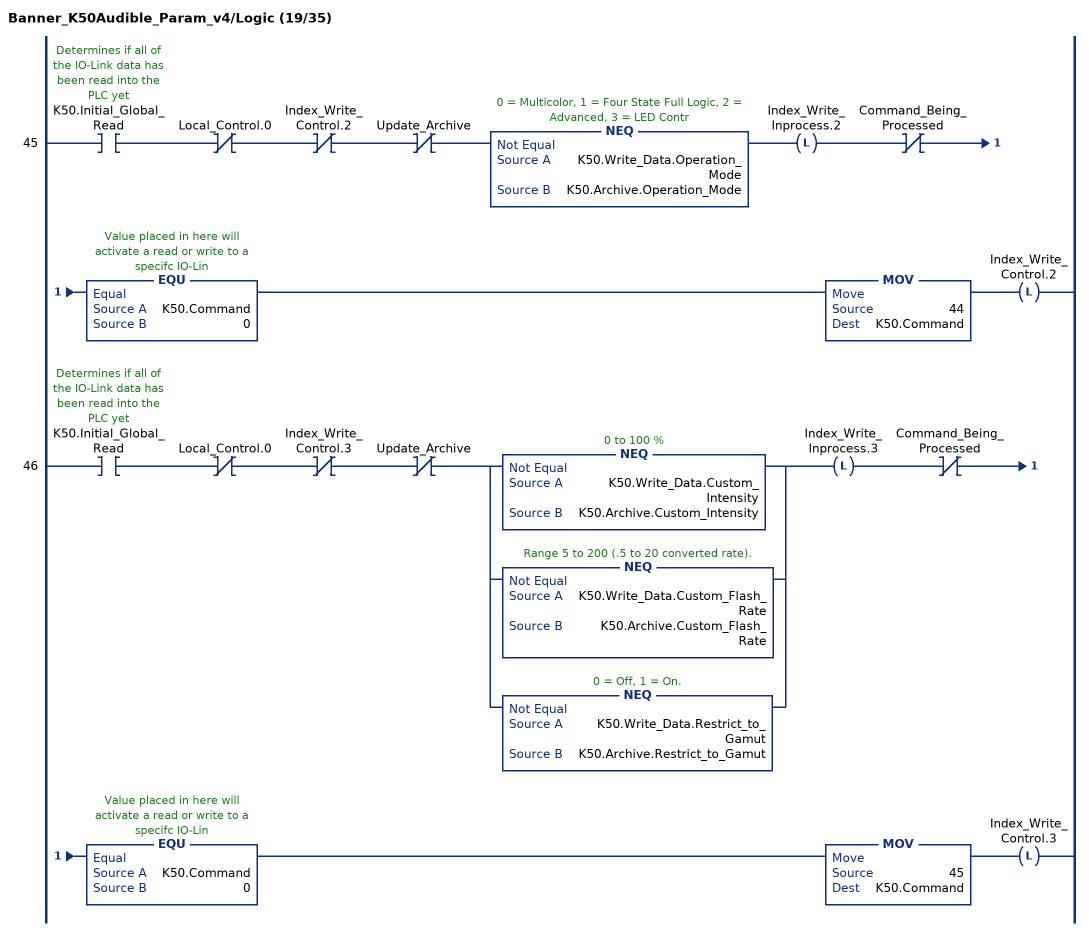
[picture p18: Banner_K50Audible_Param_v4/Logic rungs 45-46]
   45: XIC(K50.Initial_Global_Read)XIO(Local_Control.0)XIO(Index_Write_Control.2)XIO(Update_Archive)NEQ(K50.Write_Data.Operation_Mode,K50.Archive.Operation_Mode)OTL(Index_Write_Inprocess.2)XIO(Command_Being_Processed)EQU(K50.Command,0)MOV(44,K50.Command)OTL(Index_Write_Control.2);
   46: XIC(K50.Initial_Global_Read)XIO(Local_Control.0)XIO(Index_Write_Control.3)XIO(Update_Archive)[NEQ(K50.Write_Data.Custom_Intensity,K50.Archive.Custom_Intensity) ,NEQ(K50.Write_Data.Custom_Flash_Rate,K50.Archive.Custom_Flash_Rate) ,NEQ(K50.Write_Data.Restrict_to_Gamut,K50.Archive.Restrict_to_Gamut) ]OTL(Index_Write_Inprocess.3)XIO(Command_Being_Processed)EQU(K50.Command,0)MOV(45,K50.Command)OTL(Index_Write_Control.3);
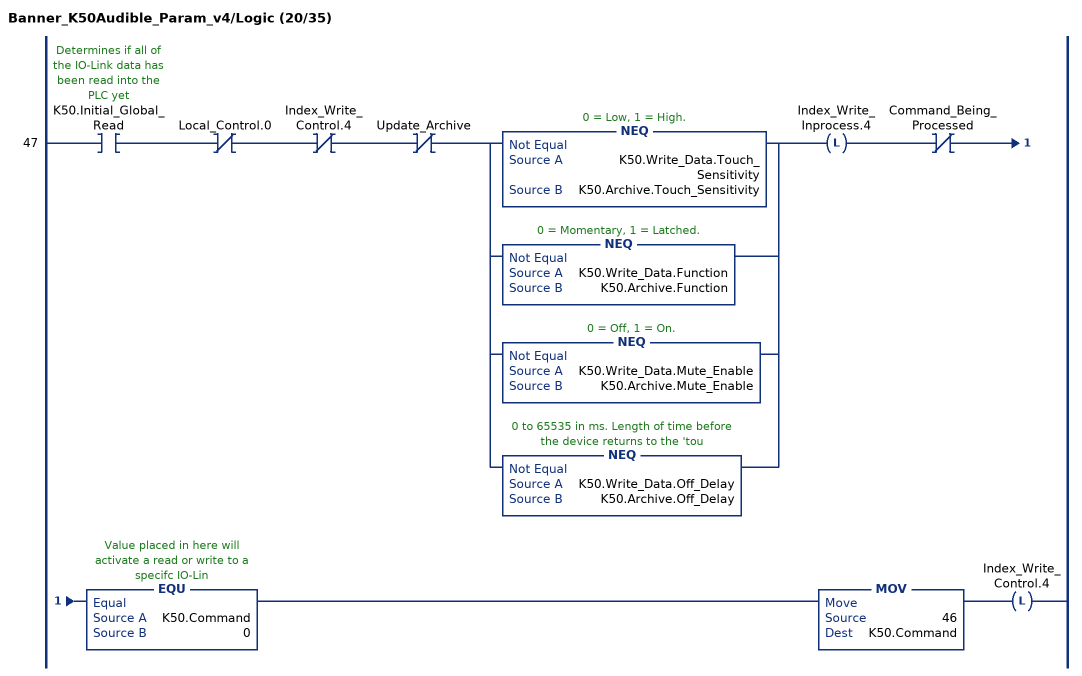
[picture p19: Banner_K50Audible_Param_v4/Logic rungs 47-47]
   47: XIC(K50.Initial_Global_Read)XIO(Local_Control.0)XIO(Index_Write_Control.4)XIO(Update_Archive)[NEQ(K50.Write_Data.Touch_Sensitivity,K50.Archive.Touch_Sensitivity) ,NEQ(K50.Write_Data.Function,K50.Archive.Function) ,NEQ(K50.Write_Data.Mute_Enable,K50.Archive.Mute_Enable) ,NEQ(K50.Write_Data.Off_Delay,K50.Archive.Off_Delay) ]OTL(Index_Write_Inprocess.4)XIO(Command_Being_Processed)EQU(K50.Command,0)MOV(46,K50.Command)OTL(Index_Write_Control.4);
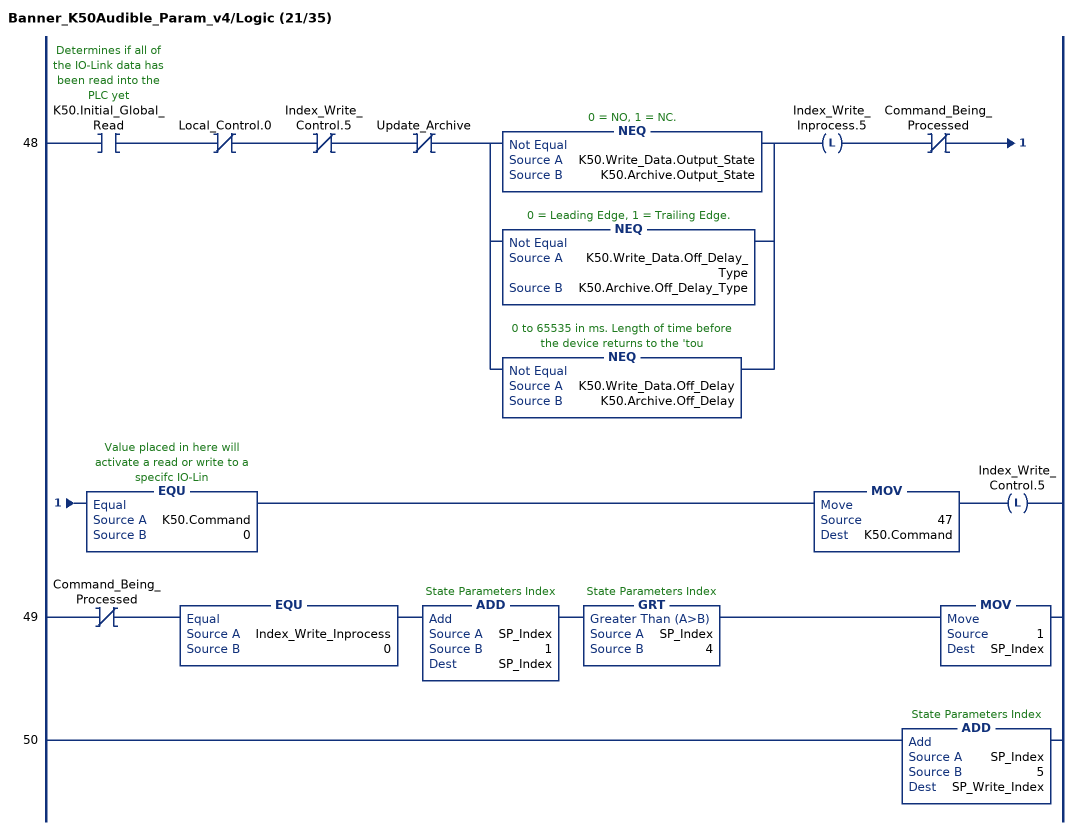
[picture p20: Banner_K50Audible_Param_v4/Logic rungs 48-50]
   48: XIC(K50.Initial_Global_Read)XIO(Local_Control.0)XIO(Index_Write_Control.5)XIO(Update_Archive)[NEQ(K50.Write_Data.Output_State,K50.Archive.Output_State) ,NEQ(K50.Write_Data.Off_Delay_Type,K50.Archive.Off_Delay_Type) ,NEQ(K50.Write_Data.Off_Delay,K50.Archive.Off_Delay) ]OTL(Index_Write_Inprocess.5)XIO(Command_Being_Processed)EQU(K50.Command,0)MOV(47,K50.Command)OTL(Index_Write_Control.5);
   49: XIO(Command_Being_Processed)EQU(Index_Write_Inprocess,0)ADD(SP_Index,1,SP_Index)GRT(SP_Index,4)MOV(1,SP_Index);
   50: ADD(SP_Index,5,SP_Write_Index);
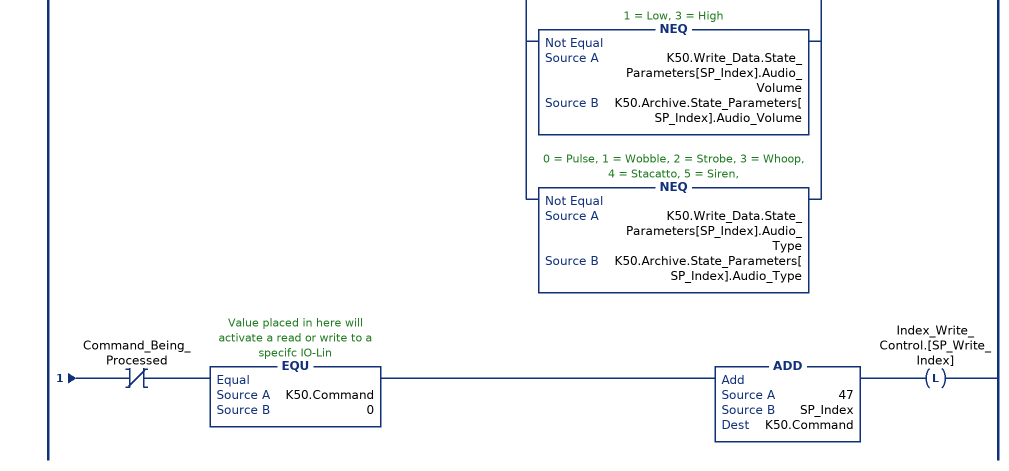
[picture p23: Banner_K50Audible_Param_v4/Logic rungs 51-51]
   51: XIC(K50.Initial_Global_Read)XIO(Local_Control.0)XIO(Index_Write_Control.[SP_Write_Index])XIO(Update_Archive)[NEQ(K50.Write_Data.State_Parameters[SP_Index].Type,K50.Archive.State_Parameters[SP_Index].Type) ,NEQ(K50.Write_Data.State_Parameters[SP_Index].Direction,K50.Archive.State_Parameters[SP_Index].Direction) ,NEQ(K50.Write_Data.State_Parameters[SP_Index].Pattern,K50.Archive.State_Parameters[SP_Index].Pattern) ,NEQ(K50.Write_Data.State_Parameters[SP_Index].Speed,K50.Archive.State_Parameters[SP_Index].Speed) ,NEQ(K50.Write_Data.State_Parameters[SP_Index].Audio_Feedback,K50.Archive.State_Parameters[SP_Index].Audio_Feedback) ,NEQ(K50.Write_Data.State_Parameters[SP_Index].Off_Delay_Type,K50.Archive.State_Parameters[SP_Index].Off_Delay_Type) ,NEQ(K50.Write_Data.State_Parameters[SP_Index].Off_Delay,K50.Archive.State_Parameters[SP_Index].Off_Delay) ,NEQ(K50.Write_Data.State_Parameters[SP_Index].Static_Sequence,K50.Archive.State_Parameters[SP_Index].Static_Sequence) ,NEQ(K50.Write_Data.State_Parameters[SP_Index].Sequence_Start_Location,K50.Archive.State_Parameters[SP_Index].Sequence_Start_Location) ,NEQ(K50.Write_Data.State_Parameters[SP_Index].Color_1,K50.Archive.State_Parameters[SP_Index].Color_1) ,NEQ(K50.Write_Data.State_Parameters[SP_Index].Color_1_Intensity,K50.Archive.State_Parameters[SP_Index].Color_1_Intensity) ,NEQ(K50.Write_Data.State_Parameters[SP_Index].Color_2,K50.Archive.State_Parameters[SP_Index].Color_2) ,NEQ(K50.Write_Data.State_Parameters[SP_Index].Color_2_Intensity,K50.Archive.State_Parameters[SP_Index].Color_2_Intensity) ,NEQ(K50.Write_Data.State_Parameters[SP_Index].Audio_Volume,K50.Archive.State_Parameters[SP_Index].Audio_Volume) ,NEQ(K50.Write_Data.State_Parameters[SP_Index].Audio_Type,K50.Archive.State_Parameters[SP_Index].Audio_Type) ]OTL(Index_Write_Inprocess.[SP_Write_Index])XIO(Command_Being_Processed)EQU(K50.Command,0)ADD(47,SP_Index,K50.Command)OTL(Index_Write_Control.[SP_Write_Index]);
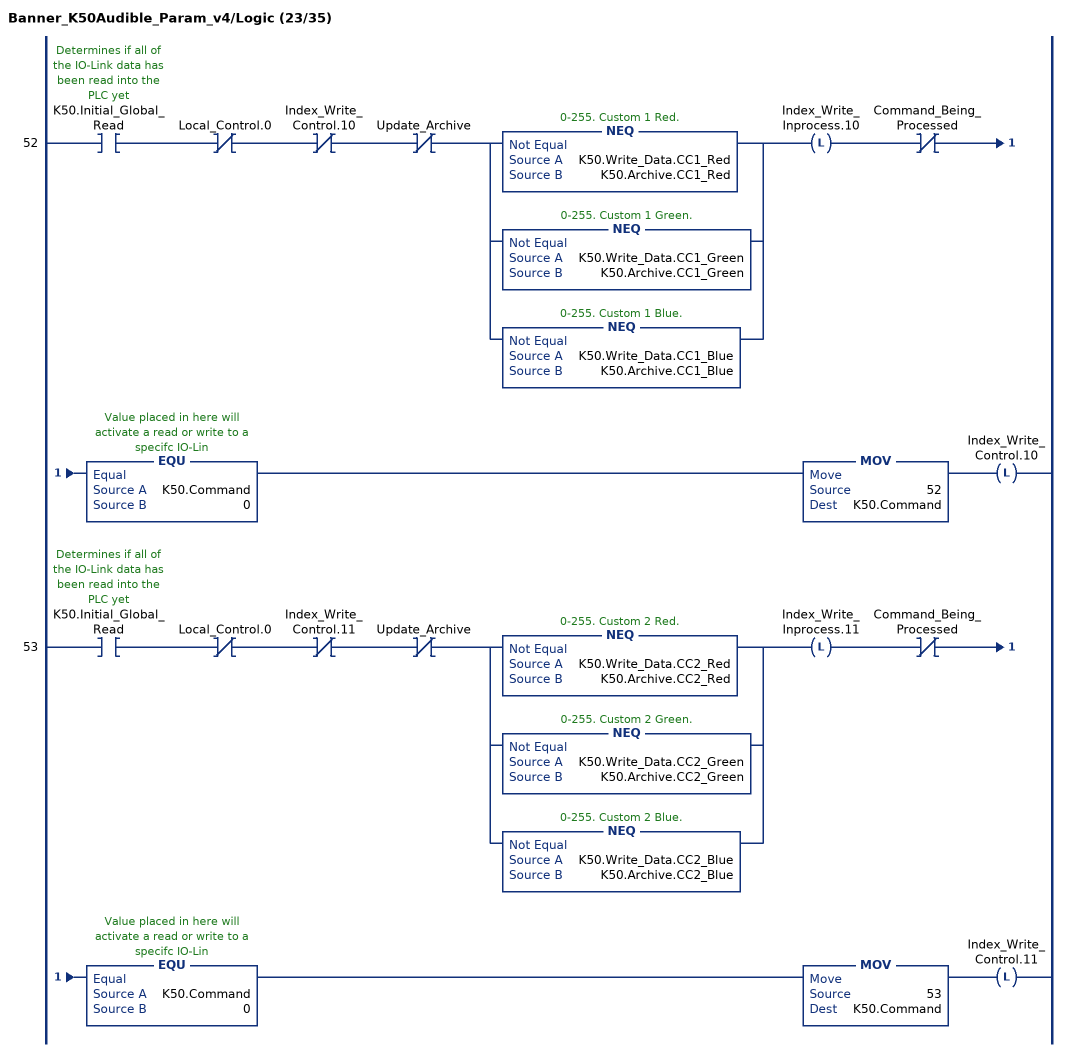
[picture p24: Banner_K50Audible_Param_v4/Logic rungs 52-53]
   52: XIC(K50.Initial_Global_Read)XIO(Local_Control.0)XIO(Index_Write_Control.10)XIO(Update_Archive)[NEQ(K50.Write_Data.CC1_Red,K50.Archive.CC1_Red) ,NEQ(K50.Write_Data.CC1_Green,K50.Archive.CC1_Green) ,NEQ(K50.Write_Data.CC1_Blue,K50.Archive.CC1_Blue) ]OTL(Index_Write_Inprocess.10)XIO(Command_Being_Processed)EQU(K50.Command,0)MOV(52,K50.Command)OTL(Index_Write_Control.10);
   53: XIC(K50.Initial_Global_Read)XIO(Local_Control.0)XIO(Index_Write_Control.11)XIO(Update_Archive)[NEQ(K50.Write_Data.CC2_Red,K50.Archive.CC2_Red) ,NEQ(K50.Write_Data.CC2_Green,K50.Archive.CC2_Green) ,NEQ(K50.Write_Data.CC2_Blue,K50.Archive.CC2_Blue) ]OTL(Index_Write_Inprocess.11)XIO(Command_Being_Processed)EQU(K50.Command,0)MOV(53,K50.Command)OTL(Index_Write_Control.11);
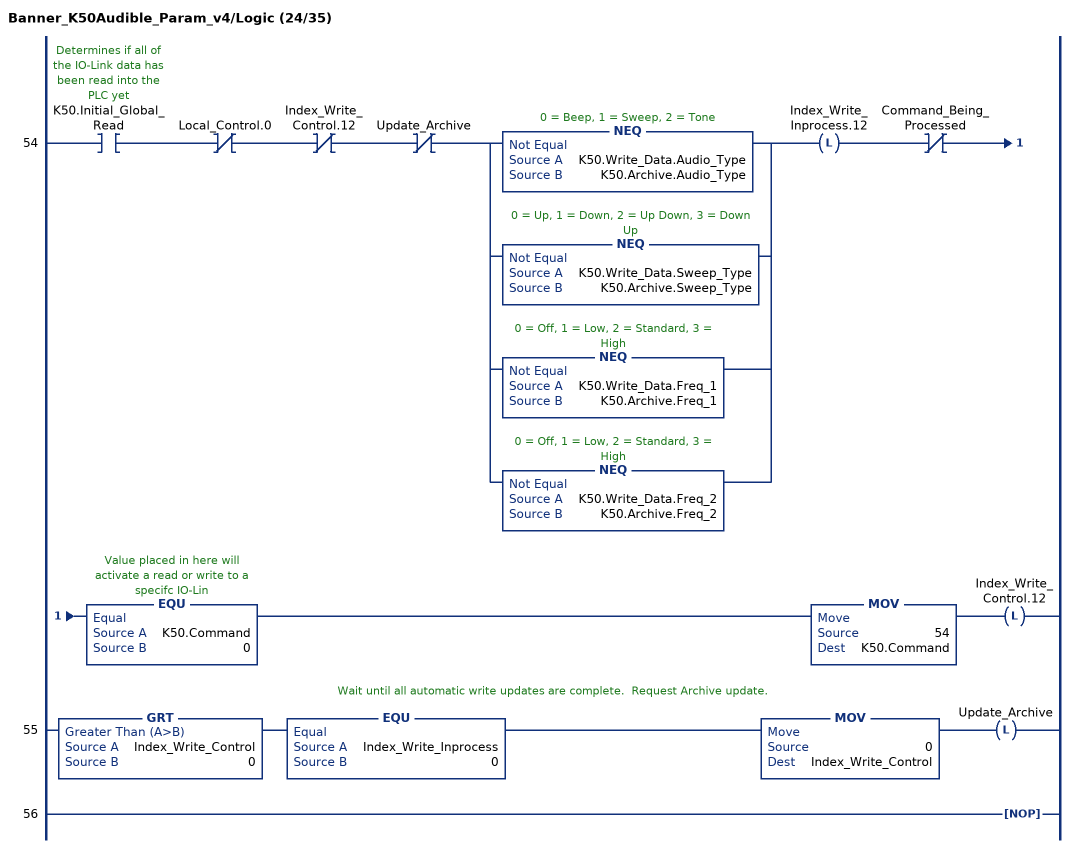
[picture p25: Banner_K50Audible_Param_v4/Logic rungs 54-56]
   54: XIC(K50.Initial_Global_Read)XIO(Local_Control.0)XIO(Index_Write_Control.12)XIO(Update_Archive)[NEQ(K50.Write_Data.Audio_Type,K50.Archive.Audio_Type) ,NEQ(K50.Write_Data.Sweep_Type,K50.Archive.Sweep_Type) ,NEQ(K50.Write_Data.Freq_1,K50.Archive.Freq_1) ,NEQ(K50.Write_Data.Freq_2,K50.Archive.Freq_2) ]OTL(Index_Write_Inprocess.12)XIO(Command_Being_Processed)EQU(K50.Command,0)MOV(54,K50.Command)OTL(Index_Write_Control.12);
   // Wait until all automatic write updates are complete.  Request Archive update.
   55: GRT(Index_Write_Control,0)EQU(Index_Write_Inprocess,0)MOV(0,Index_Write_Control)OTL(Update_Archive);
   56: NOP();
